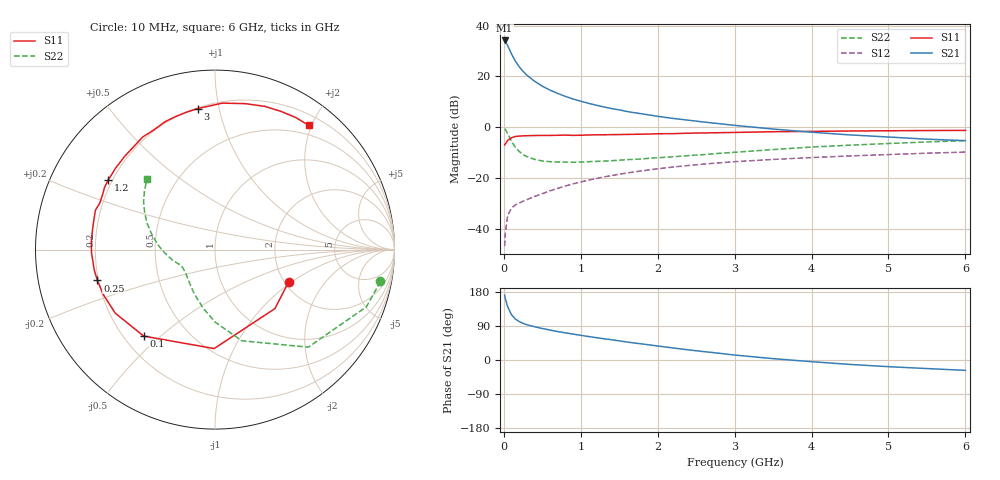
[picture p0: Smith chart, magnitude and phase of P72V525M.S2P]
! SIEMENS Small Signal Semiconductors
! BFP196
! Si NPN RF Bipolar Junction Transistor in SOT143
! VCE = 2.5 V  IC = 25 mA
! Common Emitter S-Parameters:  May  1996
# GHz  S  MA  R  50
!  f  S11  S21  S12  S22
! GHz  MAG  ANG  MAG  ANG  MAG  ANG  MAG  ANG
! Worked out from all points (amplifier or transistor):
!   36 points, 10 MHz to 6 GHz, reference 50 ohm
!   highest |S21| = 34.1 dB at 10 MHz (marker M1)
!   |S21| within 3 dB of that: start of sweep to 64.69 MHz
!   unconditionally stable (mu >= 1): 586.9 MHz to 3.472 GHz; 3.749 GHz to 4.043 GHz
!   at 250 MHz: K = 0.67, MSG = 25.5 dB, |S12| = -29.1 dB
!   at 1.4 GHz: K = 1.11, MAG = 11.2 dB, |S12| = -19.0 dB
!   at 6 GHz: K = 0.97, MSG = 2.2 dB, |S12| = -9.8 dB
!   S11 on the Smith chart (normalised r, x): 10 MHz: 2.10, -0.95; 100 MHz: 0.28, -0.44; 250 MHz: 0.20, -0.12; 1.2 GHz: 0.18, +0.29; 3 GHz: 0.21, +0.87; 6 GHz: 0.35, +1.96
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0.01  0.4483 -23.7  50.84 171.2  0.0046 82.2  0.939 -10.9
0.02  0.4684 -44.6  48.48 161.5  0.0087 75.1  0.9018 -20.7
0.05  0.5515 -90.5  40.26 140.3  0.0184 58.2  0.7521 -46.3
0.1  0.6245 -129.5  27.49 119.4  0.0259 46.1  0.5294 -73.6
0.15  0.659 -147.5  19.92 108.2  0.0298 43.0  0.4037 -89.9
0.2  0.6708 -158.0  15.49 101.4  0.0323 42.7  0.3339 -101.2
0.25  0.6776 -165.3  12.53 96.5  0.0352 44.0  0.2894 -110.3
0.3  0.6823 -170.5  10.55 93.1  0.0378 46.1  0.265 -117.0
0.4  0.6883 -178.6  8.007 87.7  0.0436 49.3  0.2333 -127.6
0.5  0.6908 175.8  6.428 83.2  0.0495 51.8  0.2176 -135.0
0.6  0.6913 170.6  5.369 79.0  0.0564 53.8  0.2106 -140.3
0.7  0.6952 166.0  4.622 75.0  0.0629 54.9  0.2077 -144.4
0.9  0.6922 158.0  3.596 68.4  0.0772 55.2  0.2056 -150.5
1.1  0.7061 150.7  2.956 62.0  0.0912 55.3  0.2107 -154.3
1.2  0.7105 146.9  2.717 59.0  0.0981 55.0  0.2135 -156.4
1.6  0.7233 134.2  2.042 47.5  0.1261 51.4  0.2306 -162.6
2.2  0.7489 117.1  1.492 31.8  0.1655 44.5  0.2628 -171.6
3  0.7915 96.9  1.09 13.1  0.2107 33.9  0.3225 174.4
3.5  0.817 87.2  0.923 3.6  0.2333 27.6  0.3644 166.0
4.5  0.8449 70.9  0.707 -11.7  0.2733 15.9  0.4446 151.9
5.5  0.8625 58.6  0.583 -22.6  0.3091 5.2  0.514 139.8
6  0.8669 53.0  0.546 -27.3  0.3253 -0.7  0.5447 134.0
